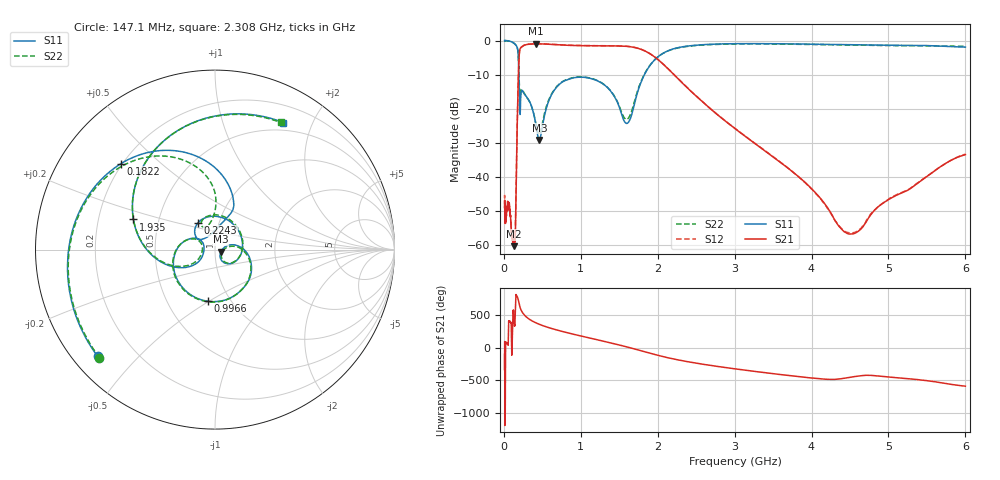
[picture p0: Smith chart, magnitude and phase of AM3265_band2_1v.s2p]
!Agilent Technologies,E8364B,MY43040894,A.07.50.67
!Agilent E8364B: A.07.50.67
!Date: Friday, May 09, 2025 07:22:32
!Correction: S11(Full 2 Port(1,2))
!S21(Full 2 Port(1,2))
!S12(Full 2 Port(1,2))
!S22(Full 2 Port(1,2))
!S2P File: Measurements: S11, S21, S12, S22:Log Frequency Sweep
# Hz S  dB  R 50
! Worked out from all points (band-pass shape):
!   3201 points, 10 MHz to 6 GHz, reference 50 ohm
!   highest |S21| = -0.97 dB at 421.9 MHz (marker M1); lowest = -60.2 dB at 127.9 MHz (marker M2)
!   |S21| within 3 dB of the highest: 200.8 MHz to 1.906 GHz (1.705 GHz wide, 162 % of centre)
!   lowest |S11| = -29.1 dB at 461.6 MHz (marker M3), VSWR 1.07, Z = 53.4 - j1.32 ohm
!   |S11| at or under -10 dB: 195.2 MHz to 1.828 GHz (1.632 GHz wide, 161 % of centre)
!   |S22| runs from -27.6 to 0.0 dB; largest |S21 - S12| = 0.0087
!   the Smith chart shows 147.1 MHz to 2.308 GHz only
!   S11 on the Smith chart (normalised r, x): 147.1 MHz: 0.07, -0.39; 182.2 MHz: 0.19, +0.38; 224.3 MHz: 0.79, +0.24; 996.6 MHz: 0.79, -0.50; 1.935 GHz: 0.36, +0.16; 2.308 GHz: 0.40, +1.60
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1e7  0.00 -7.4  -48.61 -101.5  -46.01 26.4  -0.06 -7.0
2.908064e7  -0.04 -21.0  -51.05 71.6  -50.45 73.6  -0.04 -21.0
8.439949e7  -0.22 -64.9  -51.26 38.4  -50.70 22.7  -0.25 -65.1
1.279145e8  -0.70 -110.6  -60.24 120.6  -57.89 -156.4  -0.73 -110.3
1.471268e8  -1.07 -137.7  -58.11 120.3  -56.96 -101.0  -1.10 -136.9
1.822158e8  -2.98 137.5  -16.16 30.1  -16.12 30.2  -2.89 143.2
2.243242e8  -15.08 122.8  -2.02 -148.5  -1.98 -148.5  -14.60 108.1
2.44949e8  -14.84 71.3  -1.65 169.4  -1.61 169.3  -14.62 64.5
4.219087e8  -25.46 -56.8  -0.97 14.3  -0.93 14.2  -24.96 -50.3
4.616217e8  -29.11 -20.6  -0.97 -5.5  -0.94 -5.5  -27.51 -18.7
7.123273e8  -13.03 -24.4  -1.26 -99.6  -1.23 -99.6  -12.91 -27.9
9.966268e8  -10.73 -97.5  -1.49 178.0  -1.46 178.0  -10.65 -99.9
1.307989e9  -13.02 -174.7  -1.54 93.5  -1.51 93.5  -12.96 -175.3
1.591054e9  -24.26 174.2  -1.69 13.0  -1.67 13.0  -23.10 176.0
1.935378e9  -6.29 159.7  -4.41 -96.7  -4.38 -96.7  -6.24 159.1
2.067357e9  -3.77 121.3  -6.83 -136.4  -6.81 -136.4  -3.78 121.6
2.307623e9  -1.90 61.7  -12.17 162.9  -12.14 163.0  -1.97 62.7
3.202913e9  -0.90 -91.5  -29.14 5.9  -29.13 5.9  -0.98 -91.6
3.811326e9  -1.01 -177.2  -39.52 -79.6  -39.52 -79.1  -1.08 -178.7
4.481239e9  -1.22 93.1  -56.67 -96.2  -56.28 -98.2  -1.30 91.6
5.185309e9  -1.42 1.1  -44.51 -108.1  -44.37 -108.1  -1.52 1.2
6e9  -1.93 -97.0  -33.42 132.4  -33.29 132.8  -1.69 -96.6
